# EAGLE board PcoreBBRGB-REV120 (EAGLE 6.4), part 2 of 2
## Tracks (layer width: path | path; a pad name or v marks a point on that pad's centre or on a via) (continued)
GPIO_J1_27  (via drill 0.2) (continued)
  Layer3 0.1: J9.25 60.12,5.48 59.7,5.9 52.8,5.9 51.8,6.9 51.8,12 52.05,12.25 v52.59,12.25
GPIO_J1_28  (via drill 0.2)
  Top 0.1: PCORE_.J1-28 v52.59,7.45 | v89.7,39.1 86.4,39.1 85.8,39.7 J12.5
  Layer3 0.1: v52.59,7.45 52.59,8.99 56.4,12.8 74.6,12.8 75.1,12.3 78.4,12.3 78.9,11.8 84.3,11.8 85,11.1 88.4,11.1 94,16.7 94,34.4 89.7,38.7 v89.7,39.1
GPIO_J1_29  (via drill 0.2)
  Top 0.1: PCORE_.J1-29 v52.19,11.84
  Layer3 0.1: J9.24 61.1,3.29 61.1,4.8 59.8,6.1 52.9,6.1 52,7 52,11.65 v52.19,11.84
GPIO_J1_30
  Top 0.1: PCORE_.J1-30 52.19,7.11 52.9,6.4 82.8,6.4 84.3,4.9 84.3,2.95 J9.6
GPIO_J1_31  (via drill 0.2)
  Top 0.1: PCORE_.J1-31 51.79,10.33 51.9,10.22 58.52,10.22 58.7,10.4 61.2,10.4 v62.1,9.5
  Layer3 0.1: v62.1,9.5 61.3,10.3 60.3,10.3 59.8,9.8 59.8,9.2 62.66,6.34 J9.23
GPIO_J1_32
  Top 0.1: PCORE_.J1-32 51.79,7.01 52.6,6.2 81.05,6.2 J9.7
GPIO_J1_33  (via drill 0.2)
  Top 0.1: PCORE_.J1-33 51.39,10.23 51.6,10.02 58.62,10.02 58.8,10.2 60.9,10.2 v61.6,9.5
  Layer3 0.1: v61.6,9.5 61,10.1 60.4,10.1 60,9.7 60,9.3 64,5.3 64,2.93 J9.22
GPIO_J1_34
  Top 0.1: PCORE_.J1-34 51.39,6.91 52.3,6 80.7,6 81.7,5 81.7,3.01 J9.8
GPIO_J1_35  (via drill 0.2)
  Top 0.1: PCORE_.J1-35 50.99,10.23 51.4,9.82 58.72,9.82 58.9,10 60.6,10 v61.1,9.5
  Layer3 0.1: v61.1,9.5 60.7,9.9 60.5,9.9 60.2,9.6 60.2,9.4 65.2,4.4 J9.21
GPIO_J1_36
  Top 0.1: PCORE_.J1-36 50.99,6.81 52,5.8 78.91,5.8 J9.9
GPIO_J1_37  (via drill 0.2)
  Top 0.1: PCORE_.J1-37 50.59,10.23 51.2,9.62 58.82,9.62 59,9.8 60.3,9.8 v60.6,9.5
  Layer3 0.1: J9.20 66.4,3.07 66.4,4.8 65.8,5.4 64.7,5.4 v60.6,9.5
GPIO_J1_38
  Top 0.1: PCORE_.J1-38 50.59,6.71 51.7,5.6 78.6,5.6 79.2,5 79.2,2.97 J9.10
GPIO_J1_40
  Top 0.1: PCORE_.J1-40 50.19,6.51 51.3,5.4 68.6,5.4 69.1,4.9 69.1,2.91 J9.18
GPIO_J1_42
  Top 0.1: PCORE_.J1-42 49.79,6.41 51,5.2 66.81,5.2 J9.19
HP_GND  (via drill 0.2)
  Top 0.1: v36.4,42.3 36.8,41.9 38.27,41.9 38.38,42.02 PCORE_.J2-80 | v32.3,47.8 TP1.P$1
  Bottom 0.1: v36.4,42.3 35.6,42.3 34.9,43 34.9,47 34.1,47.8 v32.3,47.8
HSYNC  (via drill 0.2)
  Top 0.1: v85.6,29.54 J12.21
  Bottom 0.1: IC10.12 84.15,27.65 85.6,29.1 v85.6,29.54
I2C_A_SCL  (via drill 0.2)
  Top 0.1: PCORE_.J1-21 v53.79,11.85 | J16.3 92.42,17.23 92.2,17 92.2,10.6 91.2,9.6 67.7,9.6 67.5,9.4 65.4,9.4 v65,9.8
  Layer2 0.1: v53.79,11.85 53.79,12.49 54.1,12.8 63.8,12.8 65,11.6 v65,9.8
  Bottom 0.1: v65,9.8 R24.2
I2C_A_SDA  (via drill 0.2)
  Top 0.1: PCORE_.J1-23 v53.39,12.25 | J16.2 92.28,18.48 92,18.2 92,10.7 91.1,9.8 v67.2,9.8
  Layer2 0.1: v53.39,12.25 53.39,12.69 53.7,13 64.8,13 67.2,10.6 v67.2,9.8
  Bottom 0.1: v67.2,9.8 R22.2
I2C_B_IRQ  (via drill 0.2)
  Top 0.1: PCORE_.J1-39 50.19,10.23 51,9.42 59.18,9.42 v59.2,9.4 | J12.49 R4.2 v81.5,11.07
  Layer2 0.1: v59.2,9.4 59.5,9.4 59.8,9.1 79.53,9.1 v81.5,11.07
I2C_B_SCL  (via drill 0.2)
  Top 0.1: PCORE_.J1-41 49.79,10.23 50.8,9.22 58.88,9.22 v59.2,8.9 | v89.9,10.9 90.3,11.3 R6.2 J12.50
  Layer2 0.1: v89.9,10.9 89.9,10.5 88.3,8.9 v59.2,8.9
I2C_B_SDA  (via drill 0.2)
  Top 0.1: PCORE_.J1-43 49.39,10.24 50.6,9.03 58.57,9.03 v59.2,8.4 | J12.48 R7.2 90.8,12.53 v90.8,11.1
  Layer2 0.1: v59.2,8.4 59.5,8.4 59.8,8.7 88.4,8.7 v90.8,11.1
JTAG_TCK  (via drill 0.2)
  Top 0.1: PCORE_.J2-18 50.79,42.09 50.5,41.8 50.5,39.2 49.1,37.8 46.8,37.8 46.1,37.1 46.1,36.9 v46.5,36.5 | v4.53,12.03 J2.4
  Layer2 0.1: v46.5,36.5 45.3,35.3 45.3,34 44.2,32.9 36.8,32.9 34.6,35.1 16.8,35.1 16.8,35 14.7,32.9 14.7,15.2 10.9,11.4 5.16,11.4 v4.53,12.03
JTAG_TDI  (via drill 0.2)
  Top 0.1: J2.8 4.73,14.57 5.4,13.9 8.1,13.9 8.42,13.58 R9.1 v8.88,12.9 | PCORE_.J2-22 49.99,42.01 50.1,41.9 50.1,39.4 48.9,38.2 46.6,38.2 45.7,37.3 45.7,36.7 v45.5,36.5
  Layer2 0.1: v45.5,36.5 45.5,36.7 45.3,36.9 44.8,36.9 44.6,36.7 44.6,33.9 44,33.3 37,33.3 34.8,35.5 16.6,35.5 14.2,33.1 14.2,18 9.1,12.9 v8.88,12.9
JTAG_TDO  (via drill 0.2)
  Top 0.1: PCORE_.J2-24 49.59,42.11 49.9,41.8 49.9,39.5 48.8,38.4 46.5,38.4 45.5,37.4 45.5,37 v45,36.5 | J2.6 4.65,13.3 v5.29,12.66
  Layer2 0.1: v45,36.5 45,34 44.1,33.1 36.9,33.1 34.7,35.3 16.7,35.3 14.4,33 14.4,17.8 9.1,12.5 5.45,12.5 v5.29,12.66
JTAG_TMS  (via drill 0.2)
  Top 0.1: PCORE_.J2-20 50.39,41.99 50.3,41.9 50.3,39.3 49,38 46.7,38 45.9,37.2 45.9,36.6 v46,36.5 | J2.2 4.15,10.76 v4.66,10.25
  Layer2 0.1: v46,36.5 46,36.7 46.2,36.9 46.7,36.9 46.9,36.7 46.9,36.3 45.6,35 45.6,34 44.3,32.7 36.7,32.7 34.5,34.9 17,34.9 14.9,32.8 14.9,15.1 11,11.2 6.3,11.2 5.7,10.6 5.01,10.6 v4.66,10.25
LCD_B0  (via drill 0.2)
  Top 0.1: PCORE_.J1-64 v45.39,7.45
  Layer3 0.1: v45.39,7.45 45.39,9.19 45.7,9.5 49.5,9.5 50.6,10.6 50.6,12.6 51.8,13.8 75.1,13.8 75.6,13.3 89.4,13.3 93.2,17.1 93.2,27 91.8,28.4 91.8,29.41 v91.76,29.45
  Bottom 0.1: v91.76,29.45 IC12.13
LCD_B1  (via drill 0.2)
  Top 0.1: PCORE_.J1-66 v44.99,7.15
  Layer3 0.1: v44.99,7.15 44.99,6.89 44.5,6.4 41.5,6.4 41.1,6.8 41.1,9.9 42.1,10.9 48.8,10.9 49.2,11.3 49.2,13.3 51.1,15.2 74.4,15.2 76.5,17.3 76.5,25.2 76.9,25.6 78.9,25.6 79.3,26 79.3,27.71 78.96,28.05 v78.4,28.05
  Bottom 0.1: v78.4,28.05 IC10.6
LCD_B2  (via drill 0.2)
  Top 0.1: PCORE_.J1-68 v44.59,7.45
  Layer3 0.1: v44.59,7.45 44.59,9.29 45,9.7 49.4,9.7 50.4,10.7 50.4,12.7 51.7,14 75.2,14 75.7,13.5 89.3,13.5 92.3,16.5 92.3,20.51 91.69,21.12 v91.09,21.12
  Bottom 0.1: v91.09,21.12 IC13.14
LCD_B3  (via drill 0.2)
  Top 0.1: PCORE_.J1-70 v44.19,7.15
  Layer3 0.1: v44.19,7.15 44.19,6.99 43.8,6.6 41.6,6.6 41.3,6.9 41.3,9.8 42.2,10.7 48.9,10.7 49.4,11.2 49.4,13.2 51.2,15 75.7,15 76.2,14.5 77.1,14.5 v78.15,15.55
  Bottom 0.1: IC11.4 79.05,15.85 79,15.9 78.5,15.9 v78.15,15.55
LCD_B4  (via drill 0.2)
  Top 0.1: PCORE_.J1-72 v43.79,7.45
  Layer3 0.1: v43.79,7.45 43.79,9.49 44.2,9.9 49.3,9.9 50.2,10.8 50.2,12.8 51.6,14.2 75.3,14.2 75.8,13.7 89.2,13.7 92.1,16.6 92.1,20.12 v91.5,20.72
  Bottom 0.1: v91.5,20.72 IC13.15
LCD_B5  (via drill 0.2)
  Top 0.1: PCORE_.J1-74 v43.39,7.15
  Layer3 0.1: v43.39,7.15 43.39,6.99 43.2,6.8 41.7,6.8 41.5,7 41.5,9.7 42.3,10.5 49,10.5 49.6,11.1 49.6,13.1 51.3,14.8 75.6,14.8 76.1,14.3 77.45,14.3 v78.7,15.55
  Bottom 0.1: v78.7,15.55 78.98,15.55 79.08,15.45 IC11.3
LCD_B6  (via drill 0.2)
  Top 0.1: PCORE_.J1-76 v42.99,7.45
  Layer3 0.1: v42.99,7.45 42.99,9.59 43.5,10.1 49.2,10.1 50,10.9 50,12.9 51.5,14.4 75.4,14.4 75.9,13.9 89.1,13.9 91.9,16.7 91.9,19.52 v91.1,20.32
  Bottom 0.1: v91.1,20.32 IC13.16
LCD_B7  (via drill 0.2)
  Top 0.1: PCORE_.J1-78 v42.59,7.15
  Layer3 0.1: v42.59,7.15 42.59,9.79 43.1,10.3 49.1,10.3 49.8,11 49.8,13 51.4,14.6 75.5,14.6 76,14.1 78,14.1 v78.5,14.6
  Bottom 0.1: v78.5,14.6 78.55,14.6 79,15.05 IC11.2
LCD_DE  (via drill 0.2)
  Top 0.1: PCORE_.J1-56 v46.99,7.45
  Layer3 0.1: v46.99,7.45 46.99,8.79 47.3,9.1 49.7,9.1 51,10.4 51,12.4 52,13.4 74.9,13.4 75.4,12.9 79.09,12.9 v79.36,12.63
  Bottom 0.1: v79.36,12.63 IC11.1
LCD_G0  (via drill 0.2)
  Top 0.1: PCORE_.J1-65 v44.99,12.15
  Layer3 0.1: v78.7,28.45 77.28,28.45 75.7,26.87 75.7,17.7 74,16 50.7,16 47.8,13.1 45.8,13.1 44.99,12.29 v44.99,12.15
  Bottom 0.1: v78.7,28.45 IC10.7
LCD_G1  (via drill 0.2)
  Top 0.1: PCORE_.J1-67 v44.59,11.85
  Layer2 0.1: v44.59,11.85 44.59,14.09 45.8,15.3 76.5,15.3 76.9,14.9 77.2,14.9 77.3,15 90.8,15 92.3,16.5 92.3,21.9 92,22.2 92,24.7 90.7,26 90.7,29.45 v91.1,29.85
  Bottom 0.1: v91.1,29.85 IC12.12
LCD_G2  (via drill 0.2)
  Top 0.1: PCORE_.J1-69 v44.19,12.15
  Layer2 0.1: v44.19,12.15 44.19,13.99 45.7,15.5 76.8,15.5 v77,15.3
  Bottom 0.1: v77,15.3 77,16.1 77.95,17.05 IC11.7
LCD_G3  (via drill 0.2)
  Top 0.1: PCORE_.J1-71 v43.79,11.85
  Layer2 0.1: v43.79,11.85 43.79,13.89 45.6,15.7 77.1,15.7 77.6,15.2 90.7,15.2 92.1,16.6 92.1,21.8 v91.58,22.32
  Bottom 0.1: v91.58,22.32 IC13.11
LCD_G4  (via drill 0.2)
  Top 0.1: PCORE_.J1-73 v43.39,12.15
  Layer2 0.1: v43.39,12.15 43.39,13.79 45.5,15.9 77.4,15.9 v77.6,15.7
  Bottom 0.1: v77.6,15.7 77.6,16.25 78,16.65 IC11.6
LCD_G5  (via drill 0.2)
  Top 0.1: PCORE_.J1-75 v42.99,11.85
  Layer2 0.1: v42.99,11.85 42.99,13.69 45.4,16.1 77.8,16.1 77.98,15.92 91.1,15.92 91.9,16.72 91.9,21.69 91.67,21.92 v91.1,21.92
  Bottom 0.1: v91.1,21.92 IC13.12
LCD_G6  (via drill 0.2)
  Top 0.1: PCORE_.J1-77 v42.59,12.15
  Layer2 0.1: v42.59,12.15 42.59,13.59 45.3,16.3 v78.16,16.3
  Bottom 0.1: IC11.5 78.21,16.25 v78.16,16.3
LCD_G7  (via drill 0.2)
  Top 0.1: PCORE_.J1-79 42.19,11.78 v42.12,11.85
  Layer2 0.1: v42.12,11.85 42.12,13.42 45.2,16.5 77.5,16.5 80.8,19.8 87.35,19.8 89.07,21.52 v91.5,21.52
  Bottom 0.1: v91.5,21.52 IC13.13
LCD_HSYNC  (via drill 0.2)
  Top 0.1: PCORE_.J1-58 v46.59,7.15
  Layer3 0.1: v46.59,7.15 46.59,6.89 45.9,6.2 41.4,6.2 40.9,6.7 40.9,10 42,11.1 48.7,11.1 49,11.4 49,13.4 51,15.4 74.3,15.4 76.3,17.4 76.3,25.3 76.8,25.8 78.8,25.8 79.1,26.1 79.1,27.51 78.96,27.65 v78.7,27.65
  Bottom 0.1: v78.7,27.65 IC10.5
LCD_PCLK  (via drill 0.2)
  Top 0.1: PCORE_.J1-50 v48.19,7.15
  Layer2 0.1: v48.19,7.15 48.19,10.79 49,11.6 49,13 49.4,13.4 90.7,13.4 93.3,16 93.3,22.2 93.6,22.5 93.6,24 91.7,25.9 91.7,28.71 v91.36,29.05
  Bottom 0.1: v91.36,29.05 IC12.14
LCD_R0  (via drill 0.2)
  Top 0.1: PCORE_.J1-47 v48.59,11.85
  Layer2 0.1: v48.59,11.85 48.59,13.29 48.9,13.6 90.6,13.6 93.1,16.1 93.1,22.3 93.4,22.6 93.4,23.9 91.5,25.8 91.5,28.55 91.4,28.65 91.11,28.65 91,28.76 91,29.23 91.5,29.73 91.5,30.15 v91.4,30.25 91.45,30.25
  Bottom 0.1: v91.4,30.25 IC12.11
LCD_R1  (via drill 0.2)
  Top 0.1: PCORE_.J1-49 v48.19,12.15
  Layer3 0.1: v78.4,28.85 78.25,28.85 78.1,28.7 77.2,28.7 75.5,27 75.5,17.8 73.9,16.2 50.6,16.2 47.7,13.3 45.7,13.3 44.9,12.5 42.1,12.5 41.7,12.1 41.7,11.6 42,11.3 48.01,11.3 48.19,11.48 v48.19,12.15
  Bottom 0.1: IC10.8 v78.4,28.85
LCD_R2  (via drill 0.2)
  Top 0.1: PCORE_.J1-51 v47.79,11.85
  Layer2 0.1: v47.79,11.85 47.79,13.19 48.4,13.8 90.5,13.8 92.9,16.2 92.9,22.4 93.2,22.7 93.2,23.8 91.12,25.88 v91.12,28.25
  Bottom 0.1: v91.12,28.25 IC12.16
LCD_R3  (via drill 0.2)
  Top 0.1: PCORE_.J1-53 v47.39,12.15
  Layer3 0.1: v78.2,26.3 77.9,26.6 76.7,26.6 76.1,26 76.1,17.5 74.2,15.6 50.9,15.6 48,12.7 47.6,12.7 47.39,12.49 v47.39,12.15
  Bottom 0.1: v78.2,26.3 78.2,27 78.45,27.25 IC10.4
LCD_R4  (via drill 0.2)
  Top 0.1: PCORE_.J1-55 v46.99,11.85
  Layer2 0.1: v46.99,11.85 46.99,13.09 47.9,14 90.4,14 92.7,16.3 92.7,22.51 92.79,22.6 v92.79,23.12
  Bottom 0.1: v92.79,23.12 IC13.9
LCD_R5  (via drill 0.2)
  Top 0.1: PCORE_.J1-57 v46.59,12.15
  Layer3 0.1: v78.6,26.84 76.63,26.84 75.9,26.11 75.9,17.6 74.1,15.8 50.8,15.8 47.9,12.9 47,12.9 46.59,12.49 v46.59,12.15
  Bottom 0.1: v78.6,26.84 IC10.3
LCD_R6  (via drill 0.2)
  Top 0.1: PCORE_.J1-59 v46.19,11.85
  Layer2 0.1: v46.19,11.85 46.19,12.89 47.5,14.2 90.3,14.2 92.5,16.4 92.5,22.62 v92.4,22.72
  Bottom 0.1: v92.4,22.72 IC13.10
LCD_R7  (via drill 0.2)
  Top 0.1: PCORE_.J1-61 v45.79,12.15
  Layer2 0.1: v45.79,12.15 45.79,13.09 47.6,14.9 v76.4,14.9
  Bottom 0.1: v76.4,14.9 76.4,15.9 77.95,17.45 IC11.8
LCD_VSYNC  (via drill 0.2)
  Top 0.1: PCORE_.J1-60 v46.19,7.45
  Layer3 0.1: v46.19,7.45 46.19,8.99 46.5,9.3 49.6,9.3 50.8,10.5 50.8,12.5 51.9,13.6 75,13.6 75.5,13.1 89.5,13.1 93.4,17 93.4,27.1 92.2,28.3 v92.2,28.65
  Bottom 0.1: v92.2,28.65 IC12.15
N$1
  Top 1.422: C1.2 H4.P$1
N$2  (via drill 0.2)
  Layer3 0.1: v68.3,7.4 68.3,6.25 J9.17
  Bottom 0.1: R22.1 R21.1 v68.3,7.4
N$3
  Top 0.127: C55.1 61.48,56.93 62.75,58.2 72.45,58.2 J15.R9
N$4  (via drill 0.2)
  Layer3 0.1: v66.1,7.4 66.5,7.4 69,4.9 69,3.4 69.4,3 71.55,3 J9.16
  Bottom 0.1: R24.1 R23.1 v66.1,7.4
N$5
  Bottom 0.4: C69.1 D8.1
  Bottom 0.406: C69.1 5.15,14.65 IC16.5
N$6
  Top 0.1: R47.2 75.85,47.6 76.75,48.5 79.25,48.5 J15.L12
N$7
  Top 0.1: R48.1 J15.R12
N$8
  Bottom 0.1: IC5.1 40.08,20.77 40.3,21 C23.1
N$9
  Bottom 0.1: IC5.3 40.38,19.48 C23.2
N$10
  Bottom 0.1: IC5.5 40.12,18.18 40.4,17.9 C24.2
N$11
  Bottom 0.1: IC5.4 40.23,18.82 40.3,18.9 C24.1
N$12  (via drill 0.2)
  Layer2 0.1: v72.87,37.15 72.87,37.03 73.1,36.8 77.4,36.8 v78.3,37.7
  Bottom 0.1: R31.1 v72.87,37.15 | v78.3,37.7 T4.1
  Bottom 0.2: T4.1 79.25,36.95 79.6,36.6 T2.3
N$13
  Bottom 0.1: C28.1 37.7,20.5 38.08,20.12 IC5.2
N$14
  Bottom 0.1: IC5.6 40.17,17.52 C29.1
N$15
  Bottom 0.1: T6.1 97.57,30.39 R39.1 97.17,32.27 97.4,32.5 J10.9@1 98.65,33.95 97.65,34.95 J10.9@2
N$16
  Bottom 0.2: D3.2 81.2,33.91 81.07,34.04 T2.1 | C38.1 80.7,35.7 81.07,35.33 T2.1 | R29.1 81.63,34.8 81.53,34.7 T2.1
N$17
  Bottom 0.1: C25.1 40.33,29.4 40.1,29.18 IC6.1
N$18
  Bottom 0.1: R37.1 76.32,38.15 77.02,38.85 T4.3
  Bottom 0.2: T4.3
N$19
  Bottom 0.2: IC8.3 R26.2
N$20
  Bottom 0.1: T3.1 75.15,39.68 74.85,39.38 C36.2 R30.1 R31.2
N$21
  Bottom 0.1: IC6.3 39.98,27.88 40.5,28.4 C25.2
N$22
  Top 0.2: R50.2 T9.1
N$23  (via drill 0.2)
  Top 0.23: PCORE_.J2-6 v53.19,41.03 | PCORE_.J2-4 v53.59,41.03 v53.6,41.02 | PCORE_.J2-2 53.99,41.1 v54.07,41.02
  Top 0.254: v54.06,41.02 v54.07,41.02
  Bottom 0.254: 53.19,40.91 53.2,40.9
  pour Bottom (no thermals): 53.07,41.28 54.19,41.28 54.36,41.11 54.36,40.48 53.98,40.1 53.98,38.68 53.9,38.6 52.09,38.6 52.04,38.65 52.04,39.82 52.87,40.65 52.87,41.08
N$24  (via drill 0.2)
  Layer2 0.25: v73.19,28.94 76.74,28.94 77.3,29.5 77.3,30.7 77,31 v76.6,31
  Bottom 0.2: IC8.4 R32.1 v76.6,31 | R33.2 R36.1 73.75,29.65 74,29.4 T5.2
  Bottom 0.254: T5.2 v73.2,28.95 v73.19,28.94
N$25  (via drill 0.2)
  Layer2 0.2: v73.75,31.9 73.75,30.77 74.53,29.99 v76.53,29.99 v76.54,30
  Bottom 0.2: R36.2 v73.75,31.9 | v76.54,30 R38.1 T5.3
N$26  (via drill 0.2)
  Top 0.254: J16.1 94.69,19.73 v95.07,19.34
  Bottom 0.254: v95.07,19.34 C71.1 L18.1
N$27  (via drill 0.2)
  Top 0.1: R71.2 28.85,61.55 29.3,62 v29.3,63.7
  Bottom 0.1: v29.3,63.7 IC9.3
N$28
  Bottom 0.1: IC6.5 40.12,26.57 40.4,26.3 C26.2
N$29
  Top 0.254: 6.9,10 6.4,9.5 7.4,9.5 6.9,10
N$30
  Bottom 0.1: IC6.4 40.23,27.23 40.3,27.3 C26.1
N$31
  Bottom 0.1: IC6.2 38.19,28.52 37.86,28.85 C31.1
N$32
  Bottom 0.1: IC6.6 40.23,25.93 40.9,25.25 C32.1
N$33
  Bottom 0.2: L11.1 C45.2 36.11,64.45 R42.2
N$34
  Top 0.1: R11.1 J2.7
N$35
  Bottom 0.2: L10.1 C44.2 R41.1
N$36  (via drill 0.3)
  other vias: 1.3,37.1 2.1,37.1 2.9,37.1 3.7,37.1 4.5,37.1 5.3,37.1 6.1,37.1 1.3,36.3 2.1,36.3 2.9,36.3 3.7,36.3 4.5,36.3 5.3,36.3 6.1,36.3 4.5,35.5 5.3,35.5 6.1,35.5
  pour Top (no thermals): 6.2,37.6 1.2,37.6 0.8,37.2 0.8,31.5 1.1,31.2 3.9,31.2 4.1,31.4 4.1,34.7 4.4,35 6.2,35 6.6,35.4 6.6,37.2
  pour Bottom (no thermals): 1.2,37.6 0.8,37.2 0.8,32.4 1.1,32.1 3.3,32.1 3.6,31.8 3.6,30.9 3.8,30.7 7.1,30.7 7.3,30.9 7.3,37.1 6.8,37.6
N$37  (via drill 0.2 pad 0.25)
  Top 0.1: SW1.2 v7.8,70.95 8.85,70.95 9.1,70.7 10.4,70.7 10.65,70.95 SW1.4
  Bottom 0.1: v7.8,70.95 8.8,69.95 8.8,68.5 9.7,67.6 R16.1 R17.1
N$39  (via drill 0.2)
  Top 0.25: v33.82,66.34 33.82,64.37 v33.15,63.7 33.15,61.95 33.9,61.2 J11.2
  Bottom 0.2: L10.2 C49.2 v33.82,66.34 | D5.2 v33.15,63.7
N$40  (via drill 0.2)
  Top 0.25: v36.5,65.5 37.75,65.5 J11.3
  Bottom 0.2: D5.1 C50.1 L11.2 35.3,65.7 35.5,65.5 v36.5,65.5
N$41
  Top 0.127: C54.1 J15.L9
N$42
  Bottom 0.2: C47.1 IC9.4
N$43  (via drill 0.2)
  Top 0.1: v38.64,57.14 R72.2 R74.1
  Layer2 0.1: v38.64,57.14 38.64,54.24 37,52.6 v37,51.03
  Bottom 0.1: v37,51.03 IC4.1
N$44  (via drill 0.2)
  Top 0.1: R63.1 v15.4,70
  Bottom 0.1: v15.4,70 R63.1
N$45  (via drill 0.2)
  Top 0.1: v41.55,49.24 R73.2 R75.1
  Bottom 0.1: v41.55,49.24 41.55,49.42 41.37,49.6 IC4.4
N$46  (via drill 0.2)
  Top 0.25: v32.2,68 32.4,68.2 J11.4 38.1,68.25 v38.1,69.7
  Bottom 0.2: D6.2 v32.2,68 | L12.2 v38.1,69.7
N$47
  Bottom 0.2: R76.2 IC17.3
N$48
  Bottom 0.2: C72.1 IC17.4
N$49  (via drill 0.2 pad 0.25)
  Top 0.1: R49.2 5.9,17.3 5.4,17.8 | 5.4,17.8 3.87,17.8 R56.2 | T10.11 v4.3,24 | v4.9,18.3 5.4,17.8
  Layer2 0.1: v4.3,24 4.3,18.9 v4.9,18.3
N$50  (via drill 0.2)
  Top 0.2: v19.2,67.5 19.9,68.2 21.8,68.2 22.4,67.6 24,67.6 25.1,66.5 J1.1 v25.1,62.1
  Bottom 0.1: C75.+ 19.2,65.87 19.19,65.86
  Bottom 0.2: L20.1 19.19,65.86 | v19.2,67.5 C75.+
  Bottom 0.254: D11.5 23.9,61.9 24.1,62.1 v25.1,62.1 25.5,61.7 25.5,58.7 D12.2
N$51
  Bottom 0.305: IC18.1 24.9,53.8 24.6,54.1 17.4,54.1 16.6,54.9 16.6,60.8 15.56,61.84 L20.2
N$52
  Bottom 0.2: D12.1 R77.2 T14.2
N$53
  Top 0.127: R54.2 19,51.8 18.5,52.3 18.5,54.57 17.97,55.1 17.6,55.1 17.48,55.23 IC14.6
N$54
  Bottom 0.1: T13.3 IC18.4 23.8,55.6 23.9,55.7 R79.1
N$55
  Bottom 0.2: T15.3 32.25,59.7 T14.1 30.65,58.45 30.36,58.16 R77.1
N$56
  Bottom 0.2: R81.2 C80.2 R78.2 33.2,56.6 33.35,56.75 T15.1
N$57
  Top 0.406: 6.8,9.7 7,9.7
N$58  (via drill 0.2 pad 0.25)
  Top 0.1: SW1.1 v7.85,69.25 8.85,69.25 9.1,69.5 10.3,69.5 10.55,69.25 SW1.3
  Bottom 0.1: R18.2 8.6,67.7 7.85,68.45 v7.85,69.25
N$63  (via drill 0.2)
  Top 0.1: v16.8,70 R65.1
  Bottom 0.1: R65.1 v16.8,70
N$64
  pour Top (no thermals): 23.7,49.2 23.7,50 23.2,50.5 21.6,50.5 21.5,50.6 21.5,55.8 21.6,55.9 23.4,55.9 24.1,55.2 24.1,50 23.9,49.8 23.9,49.2
N$65
  pour Top (no thermals): 24.9,49.2 24.9,49.9 25.5,50.5 27.1,50.5 27.3,50.7 27.3,55.7 27.1,55.9 25.4,55.9 24.6,55.1 24.6,49.9 24.7,49.8 24.7,49.2
N$66  (via drill 0.2)
  Top 0.1: v14,70 R67.1
  Bottom 0.1: R67.1 v14,70
N$67
  Top 0.1: IC15.6 21.88,46.58 R51.2
  Top 0.161: R51.2
N$68
  Top 0.2: R52.2 23.1,46 23.6,46 23.8,46.2 IC15.7
N$69
  Bottom 0.254: L4.1 C20.2 C18.+ 33.2,50.3 36.99,46.51 IC4.8
N$70
  Bottom 0.25: 41.8,45.7 42,45.9 42,49 42.8,49.8 44.1,49.8 44.6,50.3 C19.+
  Bottom 0.254: L5.1 C21.2 C19.+ | 41.8,45.7 41.3,45.7 40.8,45.2
  Bottom 0.4: 40.8,45.2 IC4.5
N$71
  Top 0.2: IC2.17 R14.2
N$72
  Top 0.2: IC15.10 25.3,45.98 | R58.2 25.3,45.98 | 25.3,45.98 25.78,45.5 25.8,45.5 25.82,45.48 R57.1
N$73
  Top 0.2: R13.2 33.25,56.2 33.7,55.75 IC2.13
N$74
  Top 0.161: IC2.21 35.85,50.55 35.95,50.45 C6.2 BQ1.3
N$75
  Top 0.127: C64.1 R59.1
N$76
  Top 0.1: IC14.2 18.12,59.42 18.43,59.73 C63.1
N$77
  Top 0.161: IC2.22 36.35,52.25 37.35,51.25 C5.2 38,48.6 BQ1.1
N$78
  Top 0.1: T9.3 16.72,60.85 R53.2 IC14.3
N$79
  Top 0.127: IC14.8 18.77,55.02 R55.2
N$84
  Top 0.1: IC14.1 18.77,59.48 18.9,59.6 19.3,59.6 19.41,59.71 R59.2
N$85
  Top 0.127: IC14.7 18.12,55.27 18.8,54.6 18.8,54.05 R60.1 R61.2
N$86
  Top 0.2: IC2.14 R12.2
N$87
  Top 0.1: IC2.24 37.35,52.25 37.65,51.95 40.85,51.95 R15.2
N$88  (via drill 0.2)
  Top 0.2: v35.85,57.1 IC2.10
  Bottom 0.2: C11.1 C8.1 35.74,57.21 v35.85,57.1
N$89
  Top 0.1: IC2.23 36.85,52.15 37.25,51.75 40.15,51.75 C14.1
N$90
  pour Top (no thermals): 17,56.3 16.7,56.3 15.6,55.2 15.6,50 16.3,49.3 18,49.3 18.2,49.5 18.2,54.6 18,54.8 17.4,54.8 17,55.2
N$120
  Top 0.2: T7.1 76.16,32.06 76.3,32.2 R43.2
N$121  (via drill 0.2)
  Top 0.2: R45.1 73.24,30.14 v72.6,29.5 | T7.3 v73.7,33.5 R44.1
  Layer2 0.2: v72.6,29.5 73.3,30.2 73.3,33.1 v73.7,33.5
N$124
  Top 0.2: T8.1 R45.2 C52.2
N$126
  Top 0.2: T8.3 77,29.16 L14.1
N$141
  Bottom 0.4: D9.1 R66.1
N$142
  Bottom 0.2: R68.1 D9.3 D10.3
PMIC_STBY  (via drill 0.2)
  Top 0.1: v43.2,41.7 PCORE_.J2-56 | v15.2,61.4 R50.1
  Bottom 0.1: v43.2,41.7 42.9,41.4 42.9,41.1 42.3,40.5 34.6,40.5 31.4,43.7 31.4,49.1 29.1,51.4 17.5,51.4 16.2,52.7 16.2,60.4 v15.2,61.4
POWERIN
  pour Top (no thermals): 5.8,53.8 8.9,53.8 9.6,54.5 9.6,56.2 8.9,56.9 1.4,56.9 0.3,55.8 0.3,40.9 0.8,40.4 4.2,40.4 4.7,40.9 4.7,52.7
R0  (via drill 0.2)
  Top 0.1: v86.4,35.89 J12.12
  Bottom 0.1: IC12.6 88.55,30.25 87.4,31.4 87.4,34.89 v86.4,35.89
R1  (via drill 0.2)
  Top 0.1: v85.6,35.89 J12.11
  Bottom 0.1: IC10.9 84.15,28.85 84.6,29.3 84.6,34.89 v85.6,35.89
R2  (via drill 0.2)
  Top 0.1: v86.4,28.25 87.98,28.25 J12.24
  Bottom 0.1: IC12.1 v86.4,28.25
R3  (via drill 0.2)
  Top 0.1: v85.6,27 J12.25
  Bottom 0.1: IC10.13 85.35,27.25 v85.6,27
R4  (via drill 0.2)
  Top 0.1: v86.4,27 J12.26
  Bottom 0.1: IC13.8 88.18,23.12 87.7,23.6 87.7,25.7 v86.4,27
R5  (via drill 0.2)
  Top 0.1: v85.6,25.73 J12.27
  Bottom 0.1: IC10.14 84.48,26.85 v85.6,25.73
R6  (via drill 0.2)
  Top 0.1: v86.4,25.73 J12.28
  Bottom 0.1: IC13.7 88.08,22.72 87.3,23.5 87.3,24.83 v86.4,25.73
R7  (via drill 0.2)
  Top 0.1: v85.6,24.46 J12.29
  Bottom 0.1: IC11.9 82.75,17.45 83.9,18.6 83.9,22.76 v85.6,24.46
RTS_C_RS232
  Bottom 0.1: IC6.7 36.17,25.27 34.7,23.8 31.6,23.8 30.8,24.6 30.8,26.9 30.2,27.5 26.27,27.5 J8.4
RXA  (via drill 0.2)
  Top 0.1: J6.3 24.04,14.34 25.2,15.5 29.7,15.5 31.2,17 31.2,18.52 v31.5,18.82
  Bottom 0.1: v31.5,18.82 IC5.13
RXB
  Bottom 0.1: IC5.8 36.12,16.23 35.3,15.4 28.5,15.4 25.1,18.8 25.1,22.21 J7.3
RXD_C_RS232
  Bottom 0.1: IC6.13 34.38,27.23 34.71,26.9 34.71,24.41 34.5,24.2 31.8,24.2 31.2,24.8 31.2,27.1 30.4,27.9 26.5,27.9 25.4,29 25.4,30.91 J8.3
SD_A_CD  (via drill 0.2)
  Top 0.1: PCORE_.J2-34 v47.59,41.75
  Layer3 0.1: v47.59,41.75 47.59,41.31 49.3,39.6 80.3,39.6 80.8,40.1 80.8,43.2 81.6,44 91,44 93,46 94.2,46 94.8,45.4 94.8,32.57 95.67,31.7 v95.67,29.85
  Bottom 0.1: v95.67,29.85 T6.3
SD_A_CLK  (via drill 0.2)
  Top 0.1: v93.64,41.65 C37.1 94.15,41.65 94.5,42 94.5,45.1 94.2,45.4 v93.4,45.4 | PCORE_.J2-38 v46.79,41.75
  Layer3 0.1: v46.79,41.75 46.79,41.31 47,41.1 47.2,41.1 49.1,39.2 80.5,39.2 81.2,39.9 81.2,43 81.8,43.6 91.2,43.6 93,45.4 v93.4,45.4
  Bottom 0.1: v93.64,41.65 J10.5
SD_A_CMD  (via drill 0.2)
  Top 0.1: R28.1 v93.65,39.4 | PCORE_.J2-36 v47.19,41.45
  Layer3 0.1: v47.19,41.45 47.19,41.41 49.2,39.4 80.4,39.4 81,40 81,43.1 81.7,43.8 91.1,43.8 93.1,45.8 94.1,45.8 94.6,45.3 94.6,40.35 v93.65,39.4
  Bottom 0.1: v93.65,39.4 94.7,39.4 J10.3
SD_A_DAT0  (via drill 0.2)
  Top 0.1: v93.65,43.85 R27.1 v92.05,43.85 | 46.6,40.8 v46.8,40.8 46.4,40.8 46.2,41 46.2,41.7 46.39,41.89 PCORE_.J2-40
  Layer3 0.1: v46.8,40.8 47.2,40.8 49,39 80.6,39 81.4,39.8 81.4,42.9 81.9,43.4 91.6,43.4 v92.05,43.85
  Bottom 0.1: v93.65,43.85 J10.7
SD_A_DAT1  (via drill 0.2)
  Top 0.1: PCORE_.J2-42 45.99,40.91 46.5,40.4 v47.1,40.4 46.7,40.4
  Layer3 0.1: v47.1,40.4 47.3,40.4 48.9,38.8 80.7,38.8 81.6,39.7 81.6,42.8 82,43.2 92,43.2 93.3,44.5 93.3,44.62 v93.63,44.95
  Bottom 0.1: v93.63,44.95 J10.8
SD_A_DAT2  (via drill 0.2)
  Top 0.1: PCORE_.J2-44 45.59,41.91 45.79,41.71 45.79,40.81 46.6,40 v46.8,40
  Layer3 0.1: v46.8,40 47.4,40 48.8,38.6 84,38.6 84.9,37.7 v89.6,37.7
  Bottom 0.1: v89.6,37.7 89.5,37.7 89.3,37.5 89.3,36.9 89.5,36.7 91.8,36.7 92.8,37.7 93.4,37.7 93.85,37.25 J10.1
SD_A_DAT3  (via drill 0.2)
  Top 0.1: v47.1,39.6 46.7,39.6 45.59,40.71 45.59,41.61 45.19,42.01 PCORE_.J2-46
  Layer3 0.1: v47.1,39.6 47.5,39.6 48.7,38.4 83.9,38.4 85.2,37.1 v89.7,37.1
  Bottom 0.1: v89.7,37.1 91.8,37.1 93.05,38.35 J10.2
SD_A_DAT4  (via drill 0.2)
  Top 0.1: PCORE_.J1-1 57.79,11.48 58.01,11.7 v58.26,11.7
  Layer2 0.1: J9.33 50.93,3.3 55.7,3.3 56.1,3.7 56.1,5 58.25,7.15 58.25,10.15 57,11.4 57,12 57.2,12.2 57.76,12.2 v58.26,11.7
SD_A_DAT5  (via drill 0.2)
  Top 0.1: PCORE_.J1-2 57.79,7.53 v57.87,7.45
  Layer2 0.1: v57.87,7.45 57.87,7.07 55.5,4.7 55.47,4.7 J9.29
SD_A_DAT6  (via drill 0.2)
  Top 0.1: PCORE_.J1-3 v57.39,11.85
  Layer2 0.1: v57.39,11.85 57.39,11.31 58.45,10.25 58.45,7.05 56.3,4.9 56.3,3.6 55.8,3.1 48.59,3.1 J9.35
SD_A_DAT7  (via drill 0.2)
  Top 0.1: PCORE_.J1-4 v57.39,7.15
  Layer2 0.1: v57.39,7.15 57.39,6.89 55.8,5.3 53.53,5.3 J9.31
SD_A_RST  (via drill 0.2)
  Top 0.1: PCORE_.J2-30 v48.39,41.75
  Layer2 0.1: v79.31,30.75 78.05,30.75 76.4,32.4 76.4,34.7 74.9,36.2 72.3,36.2 72.1,36.4 72.1,40 71.9,40.2 v71.9,40.5
  Layer3 0.1: v48.39,41.75 48.39,41.11 49.5,40 71.4,40 v71.9,40.5
  Bottom 0.1: D3.3 v79.31,30.75
SD_A_VCC  (via drill 0.2)
  Top 0.2: v93,37.3 R28.2 92.4,38.4 92.2,38.6 92.2,42.6 92.45,42.85 R27.2 | PCORE_.J2-26 v49.19,41.75
  Layer3 0.2: v49.19,41.75 49.19,41.01 49.7,40.5 70.6,40.5 71.1,41 79.2,41 v79.8,40.4 | v81.4,35.8 81.4,33.5 79.7,31.8 v74.79,31.8
  Bottom 0.2: R29.2 84,35.8 84.6,36.4 92.1,36.4 v93,37.3 | v79.8,40.4 79.8,38.5 82.05,36.25 R29.2 | C41.1 C40.1 74.42,25.45 74.55,25.58 74.55,27.02 74.89,27.36 R38.2 | IC8.5 74.55,32.7 74.79,32.46 v74.79,31.8 74.9,31.69 R32.2 R38.2 | R29.2 v81.4,35.8 | 74.89,30.09 R38.2
SD_A_VSEL  (via drill 0.2)
  Top 0.1: PCORE_.J2-28 v48.79,41.45
  Layer2 0.1: v71.3,40.5 71.9,39.9 71.9,36.3 72.1,36.1 72.1,28.69 v73.14,27.65
  Layer3 0.1: v48.79,41.45 48.79,41.01 49.6,40.2 71,40.2 v71.3,40.5
  Bottom 0.1: v73.14,27.65 T5.1 74.05,27.6 R35.2
SD_A_WP  (via drill 0.2)
  Top 0.1: PCORE_.J2-32 v47.99,41.45
  Layer3 0.1: v47.99,41.45 47.99,41.21 49.4,39.8 80.2,39.8 80.6,40.2 80.6,43.3 81.5,44.2 90.9,44.2 92.9,46.2 94.3,46.2 95,45.5 95,32.7 95.9,31.8 95.9,30.2 96.1,30 96.1,29.7 95.9,29.5 95,29.5 v94.4,30.1
  Bottom 0.1: v94.4,30.1 94.33,30.1 94.11,30.32 R25.1
SPI_A_MISO  (via drill 0.2)
  Top 0.1: PCORE_.J1-16 v54.99,7.15
  Bottom 0.1: R21.2 67.8,8.6 65.77,8.6 65.57,8.8 65.57,10 65.27,10.3 55.5,10.3 54.8,9.6 54.8,7.97 54.99,7.79 v54.99,7.15
SPI_A_MOSI  (via drill 0.2)
  Top 0.1: PCORE_.J1-18 v54.59,7.45
  Bottom 0.1: v54.59,7.45 54.59,9.69 55.4,10.5 65.6,10.5 66.1,10 R23.2
SPI_A_SCLK  (via drill 0.2)
  Top 0.1: PCORE_.J1-20 v54.19,7.15
  Layer3 0.1: v54.19,7.15 54.19,6.61 54.5,6.3 59.9,6.3 61.3,4.9 61.3,3.7 62.1,2.9 63.3,2.9 63.9,2.3 63.9,1.1 64.5,0.5 76.67,0.5 J9.12
SPI_A_SS0  (via drill 0.2)
  Top 0.1: PCORE_.J1-14 v55.39,7.45
  Layer3 0.1: v55.39,7.45 55.39,9.09 56.8,10.5 61.6,10.5 64,8.1 70.7,8.1 74.1,4.7 74.1,2.99 J9.14
TXA  (via drill 0.2)
  Top 0.1: J6.5 21.5,14.3 22.9,15.7 29.6,15.7 31,17.1 31,18.97 v31.51,19.48
  Bottom 0.1: v31.51,19.48 IC5.14
TXB
  Bottom 0.1: IC5.7 36.48,16.88 35.2,15.6 28.6,15.6 25.3,18.9 25.3,23.7 24.6,24.4 22.63,24.4 J7.5
TXD_C_RS232
  Bottom 0.1: IC6.14 34.53,27.88 34.91,27.5 34.91,24.31 34.6,24 31.7,24 31,24.7 31,27 30.3,27.7 26.4,27.7 25.2,28.9 25.2,30.3 24.5,31 22.77,31 J8.5
UART_A_RXD  (via drill 0.2)
  Top 0.1: PCORE_.J1-6 v56.99,7.45
  Layer2 0.1: v56.99,7.45 56.99,6.79 55.8,5.6 41.3,5.6 40.7,6.2 40.7,11.98 v34.5,18.18
  Bottom 0.1: R2.2 IC5.12 v34.5,18.18
UART_A_TXD  (via drill 0.2)
  Top 0.1: PCORE_.J1-8 v56.59,7.15
  Layer2 0.1: v56.59,7.15 56.59,6.79 55.6,5.8 41.4,5.8 40.9,6.3 40.9,12.1 35,18 35,18.3 34.7,18.6 34.3,18.6 34.1,18.4 34.1,17.92 v34.5,17.52
  Bottom 0.1: v34.5,17.52 IC5.11
UART_B_RXD  (via drill 0.2)
  Top 0.1: PCORE_.J1-5 56.99,12.31 55.3,14 34.7,14 33.6,15.1 33.6,15.62 v34.21,16.23
  Bottom 0.1: R3.2 IC5.9 v34.21,16.23
UART_B_TXD  (via drill 0.2)
  Top 0.1: PCORE_.J1-7 56.59,12.31 55.1,13.8 34.6,13.8 33.4,15 33.4,16.08 v34.2,16.88
  Bottom 0.1: v34.2,16.88 IC5.10
UART_C_CTS  (via drill 0.2)
  Top 0.1: PCORE_.J1-9 56.19,12.31 54.9,13.6 34.5,13.6 33.2,14.9 33.2,22.5 33.8,23.1 35,23.1 35.6,23.7 35.6,26.5 34.9,27.2 34.1,27.2 33.7,26.8 33.7,25.27 v34.34,24.62
  Bottom 0.1: IC6.9 v34.34,24.62 v34.35,24.62
UART_C_RTS  (via drill 0.2)
  Top 0.1: PCORE_.J1-11 55.79,12.31 54.7,13.4 34.4,13.4 33,14.8 33,22.6 33.7,23.3 34.9,23.3 35.4,23.8 35.4,26.4 34.8,27 34.2,27 33.9,26.7 33.9,25.72 v34.34,25.27
  Bottom 0.1: IC6.10 v34.34,25.27 v34.35,25.27
UART_C_RXD  (via drill 0.2)
  Top 0.1: PCORE_.J1-13 55.39,12.31 54.5,13.2 34.3,13.2 32.8,14.7 32.8,22.7 33.6,23.5 34.8,23.5 35.2,23.9 35.2,26.3 34.9,26.6 34.37,26.6 v34.34,26.57
  Bottom 0.1: IC6.12 v34.34,26.57 v34.35,26.57
UART_C_TXD  (via drill 0.2)
  Top 0.1: PCORE_.J1-15 54.99,12.31 54.3,13 34.2,13 32.6,14.6 32.6,22.8 33.5,23.7 34.7,23.7 35,24 35,25.8 34.88,25.93 v34.35,25.93
  Bottom 0.1: IC6.11 v34.35,25.93 v34.36,25.92
UART_D_RXD  (via drill 0.2)
  Top 0.1: PCORE_.J1-17 v54.59,11.85
  Layer2 0.1: v54.59,11.85 54.59,12.04 54.95,12.4 58.2,12.4 58.65,11.95 58.65,6.85 60.1,5.4 71.69,5.4 J9.15
UART_D_TXD  (via drill 0.2)
  Top 0.1: PCORE_.J1-19 v54.19,12.24 v54.2,12.25
  Layer2 0.1: J9.13 74.03,5.6 60.2,5.6 58.85,6.95 58.85,12.05 58.3,12.6 54.55,12.6 v54.2,12.25
USB1_EN
  Top 0.1: IC2.7 37.77,56.38 | 37.77,56.38 | 37.77,56.38 37.78,56.38 38.1,56.7 38.1,58.38 38.59,58.87 R72.1
USB1_N
  Top 0.161: IC2.19 34.85,52.42 34.97,52.3 34.97,51.95 33.97,50.95 33.97,50.32 L1.2
USB1_P
  Top 0.161: IC2.20 35.35,52.42 35.23,52.3 35.23,51.85 34.23,50.85 34.23,50.32 L1.3
USB2_EN  (via drill 0.2)
  Top 0.1: R73.1 43.64,49.24 43.98,48.9 v44,48.9 | IC2.11 35.35,57.03 v35.28,57.1
  Layer3 0.1: v35.28,57.1 35,56.82 35,51.1 37.3,48.8 43.9,48.8 v44,48.9
USB-D1_N  (via drill 0.2)
  Top 0.161: J1.2 24.3,64.07 24.03,63.8 24.03,60.52 L19.3 24.03,59.98 24.03,59.4 v24.15,59.4
  Bottom 0.161: 24.03,59.4 v24.15,59.4 24.85,60.1 D11.6
USB-D1_P  (via drill 0.2)
  Top 0.161: J1.3 23.5,64.07 23.77,63.8 23.77,60.52 L19.2 23.77,59.98 23.77,59.4 v23.65,59.4
  Bottom 0.161: 23.77,59.4 v23.65,59.4 22.95,60.1 D11.4
USB_D1_N
  Top 0.161: IC2.2 38.1,53.87 43.45,53.87 44.75,52.57 45.5,52.57 45.77,52.3 L6.4
USB_D1_P
  Top 0.161: IC2.3 38.1,54.13 43.55,54.13 44.85,52.83 45.5,52.83 45.77,53.1 L6.1
USB_D2_N
  Top 0.161: IC2.4 38.1,54.87 43.75,54.87 44.25,54.37 45.68,54.37 L7.4
USB_D2_P
  Top 0.161: IC2.5 38.1,55.13 43.85,55.13 44.35,54.63 45.68,54.63 L7.1
USB_H_N  (via drill 0.2)
  Top 0.161: v42.05,41.33 41.93,41.33 41.93,40.75 41.35,40.17 35.45,40.17 33.97,41.65 33.97,48.08 L1.1 | v42.05,43.9 41.93,43.9 41.93,44.9 41.99,44.96 PCORE_.J2-61
  Bottom 0.161: v42.05,41.33 41.93,41.33 41.93,43.9 v42.05,43.9
USB_H_P  (via drill 0.2)
  Top 0.161: v41.55,41.33 41.67,41.33 41.67,40.85 41.25,40.43 35.55,40.43 34.23,41.75 34.23,48.08 L1.4 | v41.55,43.9 41.67,43.9 41.67,44.9 41.59,44.98 PCORE_.J2-63
  Bottom 0.161: v41.55,41.33 41.67,41.33 41.67,43.9 v41.55,43.9
USB_OTG_ID  (via drill 0.2)
  Top 0.1: v45.39,47.48 45.39,46.62 45.99,46.02 PCORE_.J2-41 | J1.4 22.7,57.36 v22.94,57.12
  Layer2 0.1: v22.94,57.12 23.96,56.1 29.4,56.1 33.1,52.4 33.1,49.6 35.6,47.1 37.1,45.6 44.4,45.6 45.39,46.59 v45.39,47.48
  Bottom 0.1: v22.94,57.12 D11.3
USB_OTG_N  (via drill 0.2)
  Top 0.161: 24.28,58.55 24.03,58.3 24.03,57.85 24.45,57.43 27.85,57.43 29.53,55.75 29.53,47.35 32.33,44.55 32.33,41.05 34.05,39.33 44.35,39.33 44.77,39.75 44.77,40.06 v44.65,40.18 | 24.28,58.55 24.3,58.56 | PCORE_.J2-45 45.19,44.98 45.27,44.9 45.27,43.8 v45.15,43.8 | L19.4 24.28,58.55
  Bottom 0.161: v44.65,40.18 44.77,40.3 44.77,40.65 45.27,41.15 45.27,43.8 v45.15,43.8
USB_OTG_P  (via drill 0.2)
  Top 0.161: 23.5,58.57 23.77,58.3 23.77,57.75 24.35,57.17 27.75,57.17 29.27,55.65 29.27,47.25 32.07,44.45 32.07,40.95 33.95,39.07 44.45,39.07 45.03,39.65 45.03,40.06 v45.15,40.18 | PCORE_.J2-43 45.59,44.96 45.53,44.9 45.53,43.8 v45.65,43.8 | L19.1 23.5,58.57 | 23.5,58.57 23.5,58.58
  Bottom 0.161: v45.15,40.18 45.03,40.3 45.03,40.55 45.53,41.05 45.53,43.8 v45.65,43.8
USB_OTG_VBUS  (via drill 0.2 pad 0.25)
  Top 0.2: PCORE_.J2-37 46.79,45.91 46,46.7 46,50 v45.6,50.4
  Layer3 0.2: v45.6,50.4 45.6,50.5 40.7,55.4 40.7,59.9 40,60.6 v34.3,60.6
  Bottom 0.2: C79.2 C78.2 T14.3 31.3,61.9 32.6,60.6 v34.3,60.6
USB_PWR0
  Bottom 0.305: J4.1 52.94,61.04 51.8,59.9 51.8,56.3 51.1,55.6 38.9,55.6 37.9,54.6 L4.2
USB_PWR1
  Bottom 0.305: J4.5 53,56.1 52,55.1 40.2,55.1 39.6,54.5 L5.2
USB_PWRON  (via drill 0.2)
  Top 0.1: v33.5,54.4 33.65,54.25 IC2.16 | v41.5,46.6 41.19,46.29 PCORE_.J2-65
  Layer3 0.1: v33.5,54.4 33.5,52 37.3,48.2 39.9,48.2 40.4,47.7 40.9,47.7 41.5,47.1 v41.5,46.6
USB_VBUS  (via drill 0.2)
  Top 0.2: v27.9,53.6 28.1,53.6 28.3,53.4 28.3,46.8 31,44.1 31,40.4 33.5,37.9 43.2,37.9 v43.3,37.8 | v42.9,43.9 42.39,44.41 PCORE_.J2-59
  Layer3 0.2: v43.3,37.8 43.3,39.1 43.9,39.7 43.9,42.9 v42.9,43.9
  Bottom 0.2: R82.1 27.7,53.8 v27.9,53.6
USBD0_N
  Top 0.161: L6.3 47.92,52.57 50.7,52.57 51.88,53.75 51.88,59.35 51.4,59.83 50.05,59.83 49.63,60.25 49.63,60.8 49.87,61.04 J4.2
USBD0_P
  Top 0.161: L6.2 47.92,52.83 50.6,52.83 51.62,53.85 51.62,59.25 51.3,59.57 49.95,59.57 49.37,60.15 49.37,60.8 49.13,61.04 J4.3
USBD1_N
  Top 0.161: L7.3 47.92,54.37 49.25,54.37 49.63,54.75 49.63,58.1 49.92,58.39 J4.6
USBD1_P
  Top 0.161: L7.2 47.92,54.63 49.15,54.63 49.37,54.85 49.37,58.1 49.08,58.39 J4.7
V5OUT
  Layer2 0.254: J9.40 43.4,2.8 89.53,2.8 J9.2
  Layer2 0.4: J9.40
  Bottom 0.4: J9.40 41.07,3 34.2,3 33.5,3.7 33.5,5.2 32.15,6.55 L9.1
V33OUT
  Bottom 0.4: L8.2 33.2,9.1 33.9,8.4 33.9,7.2 35.3,5.8 40.81,5.8 J9.39 43.61,3 89.4,3 90.6,4.2 J9.1
VBAT  (via drill 0.2)
  Top 0.1: PCORE_.J2-48 44.79,41.59 v43.4,40.2
  Layer2 0.1: v37.79,31.7 30.7,31.7 30.4,31.4 30.4,22.4 29.1,21.1 29.1,10.3 27.5,8.7 10.3,8.7 R68.2 v6.55,4
  Bottom 0.1: v37.79,31.7 37.79,34.59 37.8,34.6 37.8,39.4 38.3,39.9 42.9,39.9 43.2,40.2 v43.4,40.2 | R68.2 v6.55,4
VBAT_IN  (via drill 0.2)
  Layer3 0.25: J17.2 4.9,56.07 4.9,44.6 8.4,41.1 8.4,35.3 6.2,33.1 6.2,19.1 6,18.9 4.4,18.9 3.9,18.4 3.9,10.1 5.1,8.9 9.2,8.9 11.5,6.6 v11.7,6.6
  Bottom 0.25: v11.7,6.6 R66.2
VCC_COM
  pour Bottom (no thermals): 16.9,12.9 17.6,12.2 17.6,11.2 17,10.6 15.3,10.6 13.8,12.1 13.8,42.3 15,43.5 27.8,43.5 28.9,44.6 30.5,44.6 30.5,42.8 27.8,40.2 25.9,40.2 25.6,40.5 25.6,41.6 24.8,42.4 15.6,42.4 15,41.8 15,38 15.7,37.3 17.3,37.3 18,38 18,39.1 18.5,39.7 19.5,39.7 19.9,39.3 19.9,37.6 18.6,36.3 15.6,36.3 15,35.7 15,31.5 15.6,30.9 17,30.9 17.6,30.3 17.6,29.2 16.9,28.5 15.5,28.5 15.1,28 15.1,22.3 15.6,21.8 17.1,21.8 17.6,21.3 17.6,20.1 17,19.5 15.5,19.5 15.1,19.1 15.1,13.3 15.5,12.9
VDD_SDCARD  (via drill 0.2)
  Top 0.2: R34.2 C39.1 96.58,30.89 96.31,31.16 v96.31,31.51 | R70.2 75.09,37.25 v75.19,37.15
  Layer2 0.2: v76.5,41.8 75.19,40.49 v75.19,37.15
  Bottom 0.2: T3.3 74.2,42 74.4,41.8 v76.5,41.8 76.69,41.61 D4.2 D4.1 78.69,42.09 79.39,42.79 C42.1 C43.1 83.71,42.79 86.5,40 93.65,40 94.2,40.55 J10.4 96.05,40.55 96.31,40.29 v96.31,31.51 96.17,31.37 R39.2 | R37.2 v75.19,37.15
VDD_SNVS  (via drill 0.2)
  Top 0.1: R49.1 8.5,17.3 v8.8,17.6
  Top 0.2: PCORE_.J2-50 44.39,43.61 v44.19,43.81 v44.19,43.8
  Bottom 0.1: 43.9,41.2 42.8,40.1 34.4,40.1 31,43.5 31,44.8 30.9,44.9 29,44.9 27.7,43.6 14.7,43.6 13.6,42.5 13.6,22.3 11.8,20.5 9.7,20.5 9.5,20.3 9.5,18.3 v8.8,17.6
  Bottom 0.2: IC17.5 47.12,37.8 | IC17.5 46.7,37.1 46.5,36.9 44.1,36.9 43.9,37.1 43.9,41.2 43.9,43.02 44.19,43.31 v44.19,43.8 | C74.1 47.6,38.1 47.3,37.8 IC17.5
VIN  (via drill 0.2, 0.2 pad 0.25)
  Top 0.161: R51.1 22.8,47.55 23.1,47.85 23.1,48.89 23.3,49.09 IC15.5
  Top 0.2: C60.1 22.62,49.6 22.8,49.42 IC15.5 | IC15.8 v24.3,46
  Top 0.305: C62.1 IC14.4
  Top 0.4: v13.7,58.8 C61.1 C62.1 | C60.1 C59.1 v20.55,50.6 | R55.1 v20.3,55.1 | v20.8,45.5 R52.1
  Layer2 0.2: v50.35,37.7 61.5,37.7 61.8,38 69.56,38 v71.65,35.91
  Layer2 0.406: 19.4,55.72 19.4,58.3 19.1,58.6 13.9,58.6 v13.7,58.8
  Layer3 0.2: v48.74,34.96 49.51,34.96 50,35.45 50,37.35 v50.35,37.7
  Layer3 0.305: v7.9,39.2 7.9,35.4 5.65,33.15 v5.65,19.45 3.75,19.45 2.8,18.5 v2.8,17.9
  Bottom 0.2: IC8.1 C35.1 C34.1 v71.65,35.91 | v48.74,34.96 C73.1 47.44,34.96 47.2,35.2 IC17.1 46.7,35.9 46.5,36.1 44.2,36.1 44.11,36.19 R76.1
  Bottom 0.305: v5.65,19.45 C70.1 5.65,18.15 5.8,18 6,18 6.2,17.8 IC16.2 | R64.2 v2.8,17.9
  Bottom 0.4: R62.1 v25.95,44.79
  other vias: 50.75,38.05 51.15,37.7 51.55,38.05 49.95,38.05 19.2,46.6 19.7,46.6 19.7,46.1 19.7,45.6 19.7,45.1 19.7,44.6 19.2,44.6 19.2,45.1 19.2,45.6 19.2,46.1 18.7,46.1 18.7,45.6 18.7,45.1 18.7,44.6
  pour Layer2: 28.9,46.5 35.7,39.7 43.8,39.7 44.3,39.1 49.3,39.1 49.6,39.4 51.7,39.4 52.4,38.7 52.4,38.2 51.7,37.5 33.4,37.5 27.1,43.8 19.2,43.8 18,45 18,54.3 19.3,55.8 20.9,55.8 21.1,55.6 21.1,47.2 21.8,46.5
  pour Bottom (no thermals): 49.4,40.4 49.5,40.5 51.2,40.5 51.4,40.4 51.4,38.6 51.5,38.5 51.7,38.5 51.9,38.3 51.9,37.7 51.7,37.5 49.6,37.5 49.4,37.7
  pour Bottom (no thermals): 4,40.5 3.8,40.3 3.8,38.1 3.9,38 12.5,38 12.6,38.1 12.6,40.4 12.5,40.5
  pour Bottom (no thermals): 10.8,40.3 11.7,41.2 11.7,44.9 12.6,45.9 16.9,45.9 18,47 19.8,47 20.2,46.6 20.2,44.4 19.9,44.1 14.5,44.1 13.1,42.7 13.1,38.3 12.8,38 11.3,38 10.9,38.4
VLCD
  Top 0.2: J12.47 85.33,13.03 86.6,14.3 86.7,14.3 | 86.7,14.3 J12.46 | J12.17 85.68,32.08 86,32.4 86,38.2 85.77,38.43 J12.7 C53.1 | J12.17 85.72,32.08 86,31.8 86,15 86.7,14.3 | J12.17 82.18,32.08 81.98,32.28 L13.2 | L13.2 L14.2 | R46.2 80.1,35.3 80.7,34.7 80.7,32.32 L13.2
VLCD_EN  (via drill 0.2)
  Top 0.1: 83.97,41 J12.3 v82.34,40.97 | PCORE_.J1-54 v47.39,7.15
  Top 0.2: R43.1 77.7,34.4 v78.1,34
  Layer2 0.2: v78.1,34 79,34 79.9,34.9 79.9,38.53 v82.34,40.97
  Layer3 0.1: v47.39,7.15 47.39,8.69 47.6,8.9 49.8,8.9 51.2,10.3 51.2,12.3 52.1,13.2 74.8,13.2 75.3,12.7 78.6,12.7 79.1,12.2 84.5,12.2 85.2,11.5 88.2,11.5 93.6,16.9 93.6,34.2 87.6,40.2 83.11,40.2 v82.34,40.97
VSYNC  (via drill 0.2)
  Top 0.1: v86.4,29.54 J12.22
  Bottom 0.1: IC12.2 88.15,28.65 87.26,29.54 v86.4,29.54
(copper drawn outside any net)
  shapes: Bottom circle x1, Top circle x1

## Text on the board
Top: +5V | +3V3 | +3V3_CPU | PCoreBBRGB | Rev1.20 | c 2018 | fs-net.de | POWER | RESET | BOOTSEL | Top
Layer2: Layer1
Layer3: Layer2
Bottom: + | PCoreBBRGB | c 2018 | Rev1.20 | fs-net.de | Bottom
tStop: +5V | +3V3 | +3V3_CPU | PCoreBBRGB | Rev1.20 | c 2018 | fs-net.de | POWER | RESET | BOOTSEL
bStop: + | - | PCoreBBRGB | c 2018 | Rev1.20 | fs-net.de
